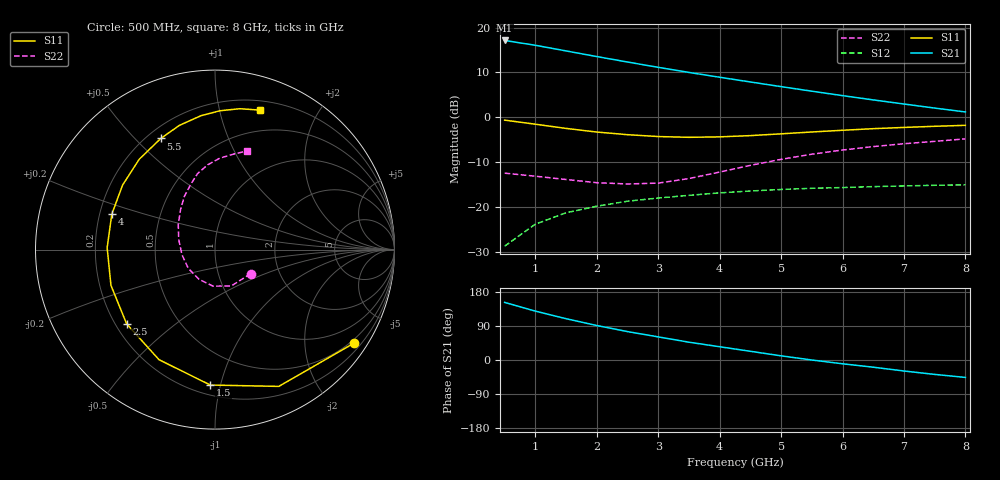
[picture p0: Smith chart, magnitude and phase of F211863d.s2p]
!ATF-21186
!S-PARAMETERS at Vds=3V  Id=70mA.  LAST UPDATED 01-30-98
# ghz s ma r 50
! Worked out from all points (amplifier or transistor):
!   16 points, 500 MHz to 8 GHz, reference 50 ohm
!   highest |S21| = 17.1 dB at 500 MHz (marker M1)
!   |S21| within 3 dB of that: start of sweep to 1.768 GHz
!   unconditionally stable (mu >= 1): 4.659 GHz to 7.911 GHz
!   at 1.5 GHz: K = 0.53, MSG = 18.0 dB, |S12| = -21.2 dB
!   at 4.5 GHz: K = 0.99, MSG = 12.1 dB, |S12| = -16.4 dB
!   at 8 GHz: K = 1.00, MSG = 8.1 dB, |S12| = -15.0 dB
!   lowest NFmin = 0.40 dB at 500 MHz
!   S11 on the Smith chart (normalised r, x): 500 MHz: 0.40, -3.23; 1.5 GHz: 0.26, -0.93; 2.5 GHz: 0.24, -0.34; 4 GHz: 0.25, +0.16; 5.5 GHz: 0.25, +0.60; 8 GHz: 0.29, +1.34
0.5  0.933 -34.0  7.181 152.0  0.037 71.0  0.24 -34.0
1  0.841 -65.0  6.348 129.0  0.065 57.0  0.222 -66.0
1.5  0.755 -92.0  5.493 109.0  0.087 46.0  0.204 -93.0
2  0.688 -117.0  4.755 91.0  0.103 38.0  0.188 -118.0
2.5  0.643 -140.0  4.135 75.0  0.117 30.0  0.182 -145.0
3  0.613 -161.0  3.607 61.0  0.127 23.0  0.186 -171.0
3.5  0.601 179.0  3.167 47.0  0.136 17.0  0.209 165.0
4  0.608 161.0  2.799 35.0  0.145 11.0  0.247 146.0
4.5  0.628 145.0  2.48 23.0  0.152 6.0  0.293 131.0
5  0.657 130.0  2.201 11.0  0.158 0.0  0.342 120.0
5.5  0.689 116.0  1.959 0.0  0.163 -5.0  0.39 110.0
6  0.72 106.0  1.748 -10.0  0.166 -11.0  0.434 103.0
6.5  0.75 96.0  1.567 -19.0  0.17 -16.0  0.474 95.0
7  0.774 88.0  1.41 -29.0  0.173 -21.0  0.51 87.0
7.5  0.797 80.0  1.271 -38.0  0.176 -26.0  0.542 79.0
8  0.817 72.0  1.151 -46.0  0.178 -31.0  0.578 72.0
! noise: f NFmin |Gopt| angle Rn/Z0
0.5  0.4  0.94  16  1.51
1  0.44  0.84  34  0.565
2  0.54  0.67  72  0.223
3  0.63  0.57  115  0.098
3.5  0.68  0.55  137  0.06
4.5  0.78  0.55  -175  0.029
5.5  0.87  0.63  -136  0.092
6  0.92  0.68  -121  0.167
7  1.01  0.78  -98  0.466
8  1.11  0.85  -78  1.089
